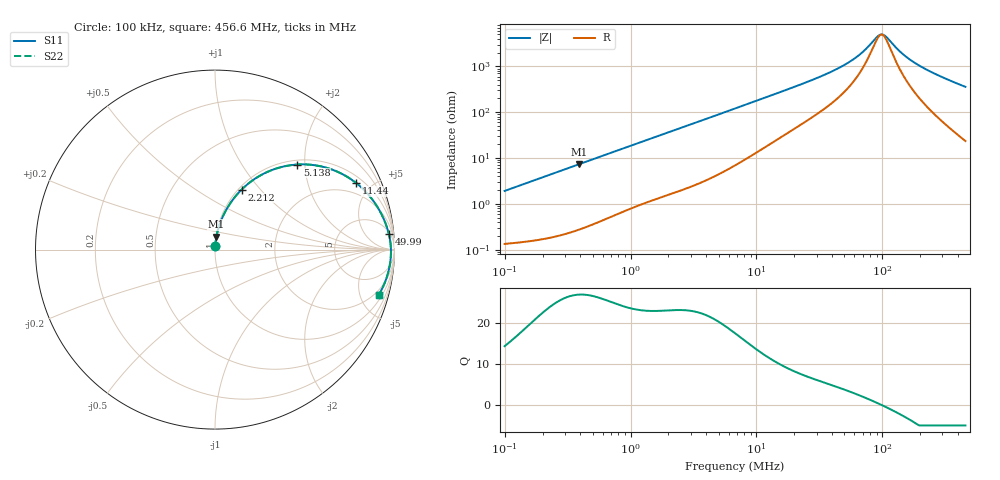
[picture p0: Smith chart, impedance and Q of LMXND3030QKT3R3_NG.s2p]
! LMXND3030QKT3R3_NG  S-PARAMETER MODEL  ( General Type )
! Model Generated by TAIYO YUDEN Corporation (https://www.yuden.co.jp/en/)
! Version 1.0
! TAIYO YUDEN Control No. 191023NI43SB-FBB
! Copyright(c) 2019 TAIYO YUDEN CO.,LTD. All Rights Reserved.
! Product Description (link to TY-COMPAS)
! https://ds.yuden.co.jp/TYCOMPAS/or/detail?pn=LMXND3030QKT3R3MNG&u=M
! Products Name : Inductors
! Characteristics :
!  Inductance : 3.3 uH , SRF(min) : 49 MHz , DC Resistance(max) : 0.0936 Ohm
!  Rated Current : Saturation :1210 mA , Temp Rise : 1230 mA (40 degC)
!  Case Size : 3.0 x 3.0 / 0.118 x 0.118 [mm/inch] , Thickness : 1.5 / 0.059 [mm/inch]
!  (Conditions: Temperature = 25 degC , DC Bias Current/Voltage = 0A / 0V)
! External Node Assignments :
!  1  o---GGG---o  2
! GND o---------o GND
! Frequency Range : 0.1MHz  -  456.598367MHz  [ 402 STEP ]
# MHz S RI R 50
! Freq[MHz].  S11 Real  S11 Imag  S21 Real  S21 Imag  S12 Real  S12 Imag  S22 Real  S22 Imag
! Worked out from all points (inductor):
!   401 points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, 100 kHz to 456.6 MHz, reference 50 ohm
!   read as one part in series: L = 3.02 uH near 104.3 kHz
!   highest Q = 26.9 at 393.3 kHz (marker M1), where L = 2.99 uH
!   self-resonance near 98.38 MHz
!   S11 on the Smith chart (normalised r, x): 100 kHz: 1.00, +0.04; 2.212 MHz: 1.03, +0.80; 5.138 MHz: 1.09, +1.83; 11.44 MHz: 1.33, +4.05; 49.99 MHz: 7, +21; 456.6 MHz: 1.47, -7.14
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0.1  0.00169 0.019  0.9983 -0.019  0.9983 -0.019  0.00169 0.019
0.393255  0.0081 0.073  0.9919 -0.073  0.9919 -0.073  0.0081 0.073
0.410178  0.00868 0.076  0.9913 -0.076  0.9913 -0.076  0.00868 0.076
0.857396  0.0306 0.1527  0.9694 -0.1527  0.9694 -0.1527  0.0306 0.1527
1.682457  0.0952 0.2724  0.9048 -0.2724  0.9048 -0.2724  0.0952 0.2724
2.212478  0.1478 0.3339  0.8522 -0.3339  0.8522 -0.3339  0.1478 0.3339
3.301465  0.268 0.4214  0.732 -0.4214  0.732 -0.4214  0.268 0.4214
5.138452  0.4584 0.474  0.5416 -0.474  0.5416 -0.474  0.4584 0.474
6.901063  0.5959 0.4626  0.4041 -0.4626  0.4041 -0.4626  0.5959 0.4626
11.44163  0.7867 0.3709  0.2133 -0.3709  0.2133 -0.3709  0.7867 0.3709
17.07324  0.878 0.2772  0.122 -0.2772  0.122 -0.2772  0.878 0.2772
27.71655  0.9369 0.1777  0.0631 -0.1777  0.0631 -0.1777  0.9369 0.1777
38.82581  0.9588 0.1215  0.0412 -0.1215  0.0412 -0.1215  0.9588 0.1215
49.9927  0.9691 0.0849  0.0309 -0.0849  0.0309 -0.0849  0.9691 0.0849
67.14138  0.9764 0.0464  0.0236 -0.0464  0.0236 -0.0464  0.9764 0.0464
94.05279  0.9801 0.0054  0.0199 -0.0054  0.0199 -0.0054  0.9801 0.0054
102.3215  0.9804 -0.00473  0.0196 0.00473  0.0196 0.00473  0.9804 -0.00473
113.6871  0.9804 -0.0175  0.0196 0.0175  0.0196 0.0175  0.9804 -0.0175
143.3337  0.979 -0.0465  0.021 0.0465  0.021 0.0465  0.979 -0.0465
188.4878  0.9744 -0.0839  0.0256 0.0839  0.0256 0.0839  0.9744 -0.0839
281.262  0.9588 -0.1488  0.0412 0.1488  0.0412 0.1488  0.9588 -0.1488
456.5984  0.9135 -0.2502  0.0865 0.2502  0.0865 0.2502  0.9135 -0.2502
